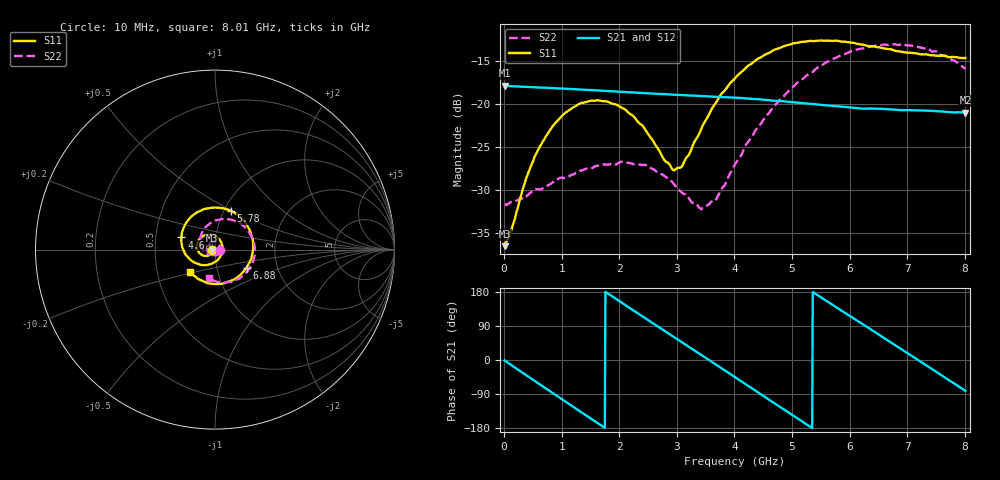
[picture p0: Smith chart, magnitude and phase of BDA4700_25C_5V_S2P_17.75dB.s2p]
!Agilent Technologies,E5071B,MY42404982,A.09.10
!Date: Mon Oct 20 13:35:11 2025
!Data & Calibration Information:
!Freq	S11:SOLT2(ON)	S21:SOLT2(ON)	S12:SOLT2(ON)	S22:SOLT2(ON)
# Hz S RI R 50
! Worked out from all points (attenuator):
!   801 points, 10 MHz to 8.01 GHz, reference 50 ohm
!   highest |S21| = -17.85 dB at 10 MHz (marker M1); lowest = -21.0 dB at 8.01 GHz (marker M2)
!   lowest |S11| = -36.5 dB at 10 MHz (marker M3), VSWR 1.03, Z = 48.5 - j0.131 ohm
!   |S11| at or under -10 dB: start of sweep to end of sweep
!   |S22| runs from -32.2 to -13.0 dB; largest |S21 - S12| = 0.00097
!   S11 on the Smith chart (normalised r, x): 10 MHz: 0.97, -0.00; 4.6 GHz: 0.68, +0.10; 5.78 GHz: 1.08, +0.49; 6.88 GHz: 1.39, -0.29; 8.01 GHz: 0.74, -0.19
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1e7  -0.0149 -0.00135  0.1281 -0.00275  0.1281 -0.00295  0.0259 -0.000872
1.5e8  -0.0165 -0.0107  0.1223 -0.0347  0.1222 -0.0347  0.0262 -0.00707
3.9e8  -0.0264 -0.0266  0.0957 -0.0821  0.0956 -0.0821  0.0209 -0.0203
6e8  -0.0424 -0.035  0.0585 -0.1106  0.0584 -0.1106  0.0127 -0.0293
1e9  -0.0816 -0.024  -0.0277 -0.1201  -0.0276 -0.1202  -0.0154 -0.0341
1.35e9  -0.101 0.0121  -0.0912 -0.0805  -0.0912 -0.0805  -0.0374 -0.0172
1.76e9  -0.0825 0.0632  -0.1195 0.000234  -0.1196 0.000285  -0.0422 0.0141
2.08e9  -0.0424 0.084  -0.0995 0.0631  -0.0996 0.0632  -0.0283 0.036
2.68e9  0.0341 0.0425  0.00495 0.1147  0.00495 0.1147  0.016 0.0364
2.93e9  0.0415 0.0022  0.0523 0.1009  0.0524 0.1007  0.027 0.0221
3.05e9  0.0386 -0.018  0.0719 0.0873  0.0715 0.0876  0.0288 0.0124
3.43e9  -0.00616 -0.0723  0.1089 0.0245  0.1089 0.0245  0.0182 -0.0165
3.69e9  -0.0571 -0.0861  0.1074 -0.0252  0.1075 -0.0255  -0.00182 -0.0281
4.01e9  -0.1255 -0.0652  0.0768 -0.0776  0.0768 -0.0774  -0.0355 -0.0268
4.6e9  -0.1868 0.0679  -0.0267 -0.1021  -0.0267 -0.1021  -0.0806 0.0375
5.35e9  -0.0486 0.2281  -0.1003 -0.000828  -0.1004 -0.00111  -0.0136 0.1528
5.78e9  0.0901 0.216  -0.0723 0.0651  -0.0721 0.0651  0.0842 0.1672
6.23e9  0.1929 0.1096  -0.007 0.094  -0.00617 0.0941  0.1818 0.1071
6.68e9  0.2055 -0.0395  0.0601 0.0715  0.0603 0.0715  0.2216 -0.00718
6.88e9  0.1762 -0.0999  0.0796 0.0468  0.0799 0.0465  0.2128 -0.0636
7.44e9  0.0206 -0.1912  0.0829 -0.0386  0.0829 -0.0387  0.1086 -0.1708
8.01e9  -0.139 -0.1233  0.0132 -0.0885  0.0133 -0.0886  -0.0361 -0.1565
